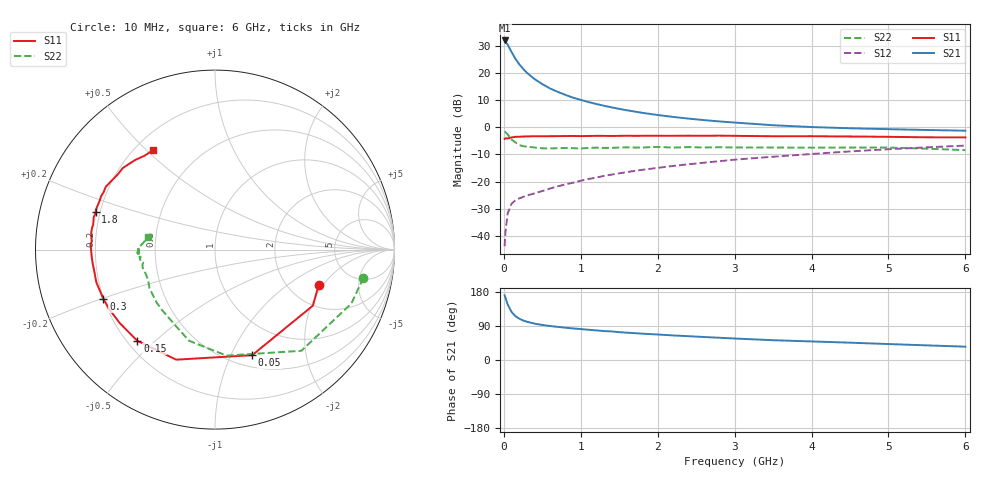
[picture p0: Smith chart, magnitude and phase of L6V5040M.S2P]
!  INFINEON TECHNOLOGIES Small Signal Semiconductors
! BFR380L3 , Si-NPN RF-Transistor in TSLP-3-1
!  Vce=0.5 V,  Ic=40 mA
! Common Emitter S-Parameters:  07. March 2005
#  GHz  S  MA  R  50
! f  S11  S21  S12  S22
! GHz  Mag  Ang  Mag  Ang  Mag  Ang  Mag  Ang
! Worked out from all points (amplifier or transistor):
!   36 points, 10 MHz to 6 GHz, reference 50 ohm
!   highest |S21| = 32.1 dB at 10 MHz (marker M1)
!   |S21| within 3 dB of that: start of sweep to 76.56 MHz
!   unconditionally stable (mu >= 1): 911.8 MHz to end of sweep
!   at 250 MHz: K = 0.54, MSG = 23.7 dB, |S12| = -25.7 dB
!   at 1.4 GHz: K = 1.07, MAG = 10.8 dB, |S12| = -17.5 dB
!   at 6 GHz: K = 1.03, MAG = 1.6 dB, |S12| = -6.7 dB
!   S11 on the Smith chart (normalised r, x): 10 MHz: 2.88, -1.82; 50 MHz: 0.63, -1.21; 150 MHz: 0.24, -0.44; 300 MHz: 0.20, -0.20; 1.8 GHz: 0.18, +0.15; 6 GHz: 0.27, +0.52
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0.01  0.6105 -18.9  40.15 170.5  0.0064 74.9  0.8415 -10.8
0.02  0.6284 -29.8  38.93 165.2  0.0114 75.1  0.8169 -21.6
0.05  0.6236 -70.6  33.5 146.4  0.0259 61.3  0.7412 -49.5
0.1  0.6502 -109.4  24.59 126.9  0.0389 47.7  0.594 -83.8
0.15  0.6674 -130.4  18.45 115.7  0.0449 42.1  0.5282 -105.9
0.2  0.6703 -142.2  14.62 109.1  0.0487 41.3  0.4723 -119.0
0.25  0.6762 -150.6  12.05 104.4  0.0519 40.7  0.4482 -131.0
0.3  0.6798 -156.1  10.17 101.0  0.0551 42.2  0.4393 -137.6
0.4  0.6857 -164.5  7.765 95.9  0.0605 44.4  0.4241 -149.3
0.5  0.6834 -170.0  6.277 92.5  0.0667 48.1  0.4099 -155.2
0.6  0.686 -173.6  5.22 89.7  0.074 51.1  0.4085 -159.5
0.7  0.688 -176.4  4.516 87.4  0.0814 53.2  0.4111 -163.3
0.8  0.6903 -179.7  3.969 85.2  0.0883 54.9  0.4157 -166.0
0.9  0.6928 177.6  3.527 83.3  0.095 56.3  0.412 -168.6
1.1  0.6929 174.0  2.929 79.8  0.1111 58.6  0.4173 -170.5
1.4  0.6928 168.6  2.338 75.4  0.1339 60.4  0.4179 -173.8
1.8  0.6979 162.3  1.854 69.5  0.1642 61.1  0.4229 -177.0
2.2  0.6978 157.3  1.557 64.8  0.1937 61.1  0.4228 -178.0
3.5  0.6846 142.0  1.093 52.2  0.2863 58.3  0.4238 179.2
4.5  0.6772 135.5  0.961 45.7  0.3592 55.3  0.4236 178.3
5.5  0.654 126.9  0.893 38.6  0.4276 50.1  0.4032 175.0
6  0.6527 121.9  0.867 35.2  0.46 47.5  0.379 169.4
